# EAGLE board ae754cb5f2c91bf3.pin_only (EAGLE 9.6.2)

Size 15.24 x 20.45 mm. Coordinates in mm from the lower left corner, seen from the top.
Outline: 12.7,0 arc90 15.24,2.54 15.24,17.91 arc90 12.7,20.45 2.54,20.45 arc90 0,17.91 0,2.54 arc90 2.54,0 12.7,0
Copper layers (1*16): Top 0.035mm / dielectric 1.5mm / Bottom 0.035mm
Design rules "default *": minimum track width 8mil, minimum drill 0.4mm, track to track 8mil, track to pad 8mil, pad to pad 8mil, via to via 8mil, smd to smd 8mil, copper to edge 20mil, drill to drill 8mil, minimum pad ring 8mil, minimum via ring 10mil, stop-mask expansion 3mil, vias tented up to drill 20mil, thermal gap 8mil

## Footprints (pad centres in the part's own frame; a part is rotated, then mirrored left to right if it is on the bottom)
1X06-CLEANBIG = drill 1.016 pad 1.778 octagon: 1 -6.35,0; 2 -3.81,0; 3 -1.27,0; 4 1.27,0; 5 3.81,0; 6 6.35,0
SOT23 = smd 1 x 1.4: 1 -0.95,-1.1; 2 0.95,-1.1; 3 0,1.1
R0805 = smd 1.1 x 1.4: 1 -1,0; 2 1,0

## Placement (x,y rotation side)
JP3  [1X06-CLEANBIG]  2.54,10.16 90 top
JP4  [1X06-CLEANBIG]  12.7,10.16 90 top
Q1  BSS138  [SOT23]  9.4,14.48 270 top
Q2  BSS138  [SOT23]  6.1,11.94 270 top
Q3  BSS138  [SOT23]  9.65,7.11 270 top
Q4  BSS138  [SOT23]  5.84,4.06 270 top
R1  10K  [R0805]  5.59,17.02 180 top
R2  10K  [R0805]  9.91,11.94 0 top
R3  10K  [R0805]  9.4,17.02 180 top
R4  10K  [R0805]  5.59,14.99 180 top
R5  10K  [R0805]  5.59,9.14 180 top
R6  10K  [R0805]  9.91,9.91 180 top
R7  10K  [R0805]  9.65,4.06 180 top
R8  10K  [R0805]  5.59,6.86 180 top
U$1  [ADAFRUIT_3.5MM]  9.4,16.26 0 bottom

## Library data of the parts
JP3 JP4 Q1-Q4 R1-R8 = adafruit
U$1 = microbuilder

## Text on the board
tPlace: 4 Bi-Directional | HV | LV | B1 | A1 | B2 | A2 | B3 | A3 | B4 | A4 | GND | GND | Level Shifters
bPlace: LV:1.8V-HV | HV:LV-10V | Works with | TTL Serial | I2C SPI | adafruit! | BSS138 FETs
